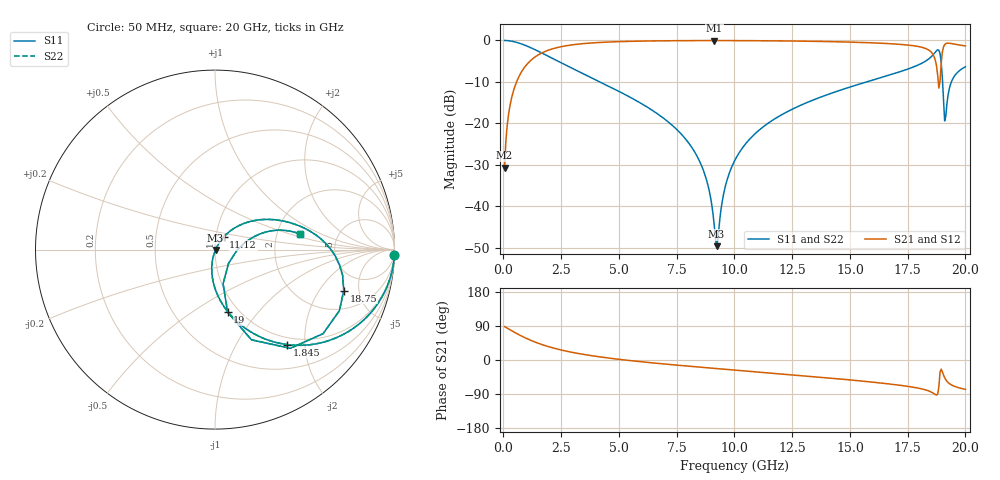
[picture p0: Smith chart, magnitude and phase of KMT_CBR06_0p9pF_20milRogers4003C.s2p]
! Data measured by Modelithics Inc. support@modelithics.com 813-866-6335
! KEMET CBR0603 0.9pF, Pad Width= 0.851mm, Pad Length= 0.64mm, Pad Gap= 0.62mm, 20mil Rogers 4003C substrate Data, January 2022
# hz S ma R 50
! 2 Port Network Data from SP1.SP block
! freq  magS11  angS11  magS21  angS21  magS12  angS12  magS22  angS22
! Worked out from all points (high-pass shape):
!   401 points, 50 MHz to 20 GHz, reference 50 ohm
!   highest |S21| = -0.03 dB at 9.127 GHz (marker M1); lowest = -30.7 dB at 50 MHz (marker M2)
!   |S21| within 3 dB of the highest: 1.655 GHz to 18.55 GHz (16.9 GHz wide, 167 % of centre); 19 GHz to end of sweep
!   lowest |S11| = -49.6 dB at 9.227 GHz (marker M3), VSWR 1.01, Z = 50.3 - j0.154 ohm
!   |S11| at or under -10 dB: 4.183 GHz to 15.71 GHz (11.53 GHz wide, 116 % of centre); 19.01 GHz to 19.39 GHz (381.4 MHz wide, 1.99 % of centre)
!   |S22| runs from -49.6 to 0.0 dB; largest |S21 - S12| = 0
!   S11 on the Smith chart (normalised r, x): 50 MHz: 1, -64; 1.845 GHz: 0.88, -1.66; 11.12 GHz: 1.09, +0.15; 18.75 GHz: 3.28, -3.46; 19 GHz: 0.89, -0.71; 20 GHz: 2.70, +0.61
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5e7  0.9996 -1.8  0.02929 88.2  0.02929 88.2  0.9996 -1.8
2.99375e8  0.9849 -10.7  0.1729 79.3  0.1729 79.3  0.9849 -10.7
5.98625e8  0.943 -20.9  0.332 69.1  0.332 69.1  0.943 -20.9
1.8455e9  0.6653 -52.7  0.745 37.2  0.745 37.2  0.6653 -52.7
3.391625e9  0.405 -74.2  0.9121 15.5  0.9121 15.5  0.405 -74.2
6.73325e9  0.1269 -98.0  0.9889 -9.2  0.9889 -9.2  0.1269 -98.0
8.429e9  0.03811 -103.8  0.9958 -18.5  0.9958 -18.5  0.03811 -103.8
8.877875e9  0.01688 -99.8  0.9963 -20.8  0.9963 -20.8  0.01688 -99.8
9.12725e9  0.005904 -78.2  0.9964 -22.1  0.9964 -22.1  0.005904 -78.2
9.227e9  0.003327 -27.3  0.9964 -22.6  0.9964 -22.6  0.003327 -27.3
9.626e9  0.01837 54.7  0.9961 -24.6  0.9961 -24.6  0.01837 54.7
1.0025e10  0.03631 57.8  0.9955 -26.6  0.9955 -26.6  0.03631 57.8
1.112225e10  0.08551 55.3  0.9921 -32.1  0.9921 -32.1  0.08551 55.3
1.336662e10  0.1896 45.0  0.9766 -43.6  0.9766 -43.6  0.1896 45.0
1.670825e10  0.3832 25.5  0.9146 -63.3  0.9146 -63.3  0.3832 25.5
1.830425e10  0.5707 8.0  0.7947 -79.4  0.7947 -79.4  0.5707 8.0
1.875312e10  0.753 -17.6  0.4875 -92.3  0.4875 -92.3  0.753 -17.6
1.890275e10  0.6921 -52.6  0.3215 -31.9  0.3215 -31.9  0.6921 -52.6
1.90025e10  0.3556 -78.6  0.7239 -31.1  0.7239 -31.1  0.3556 -78.6
1.915212e10  0.1228 -1.7  0.9166 -52.1  0.9166 -52.1  0.1228 -1.7
1.945138e10  0.3436 18.0  0.9116 -67.5  0.9116 -67.5  0.3436 18.0
2e10  0.4816 10.3  0.858 -77.6  0.858 -77.6  0.4816 10.3
